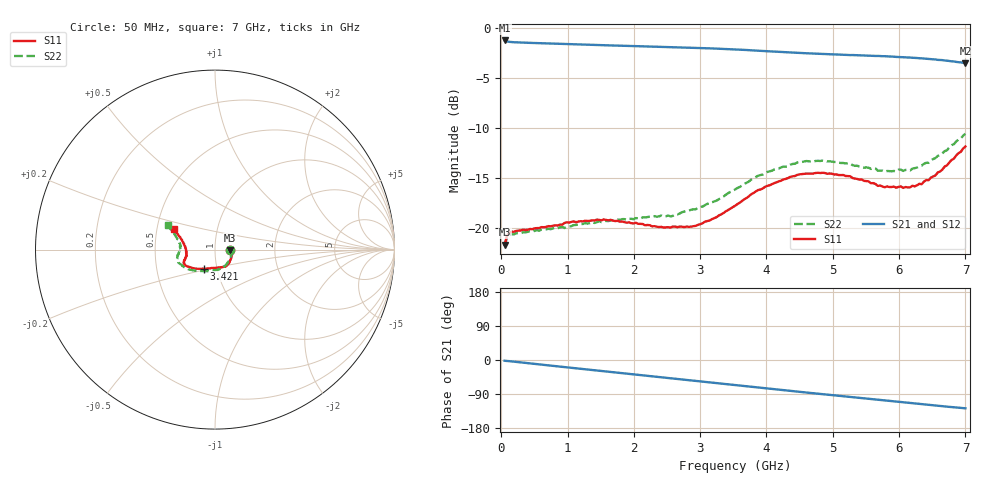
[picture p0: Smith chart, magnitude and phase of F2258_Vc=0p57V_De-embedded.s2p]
! Integrated Device Technology
! Corporate Headquarters
! 6024 Silver Creek Valley Road
! San Jose, CA 95138  USA
! Phone:  1-408-284-8200
! Toll Free:  1-800-223-1366
! Webpage:  http://www.idt.com/
! Timing and RF Division
! 515 Groton Road, Suite 102
! Westford, MA 01886-6024
! Device:  F2258
! Description: Voltage Variable RF Attenuator
! Frequency:  50.0 -  6000.00 MHz
! Package:  3x3 mm Thin QFN Plastic Package: 16 pin
! Ports:  2 RF, 2 DC
!  Pin  1  = NC
!  Pin  2  = NC
!  Pin  3  = RF2  = Port 2
!  Pin  4  = GND
!  Pin  5  = Vdd
!  Pin  6  = NC
!  Pin  7  = VCTRL
!  Pin  8  = NC
!  Pin  9  = GND
!  Pin 10  = RF1  = Port 1
!  Pin 11  = NC
!  Pin 12  = NC
!  Pin 13  = NC
!  Pin 14  = NC
!  Pin 15  = NC
!  Pin 16  = NC
! Vcntrl:  0.570 Volts
! Vdd:  +3.300 Volts
! Current:  1.106 mA
! Data:  The device was measured on a the F2258 evaluation board which has
!  individual transmission lines to the RF pins.  Data was collected
!  using a calibrated network analyzer.  The evaluation board was
!  de-embedded using a TRL calibration technique.
!  The reference plane is the edge of the package pin.
! Misc:  SN 10
!  Action Tracker AT0285
! Date Measured:  2014-12-10
! Date:  2016-01-13  MJV
! Note:
!  Integrated Device Technology supplies this data as a sample of measured
!  data at the package pin for this product.  Your particular data for this
!  product may vary.
!  Data was taken at 25 degrees C.
!  Integrated Device Technology reserves the right to change this data at anytime.
!Freq_(GHz)  S11M_(dB)  S11P_(deg)  S21M_(dB)  S21P_(deg)  S12M_(dB)  S12P_(deg)  S22M_(dB)  S22P_(deg)
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# GHz S dB R 50
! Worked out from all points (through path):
!   201 points, 50 MHz to 7 GHz, reference 50 ohm
!   highest |S21| = -1.21 dB at 50 MHz (marker M1); lowest = -3.5 dB at 7 GHz (marker M2)
!   group delay of S21, straight-line fit = 50.5 ps
!   lowest |S11| = -21.6 dB at 50 MHz (marker M3), VSWR 1.18, Z = 59 - j0.48 ohm
!   |S11| at or under -10 dB: start of sweep to end of sweep
!   |S22| runs from -21.8 to -10.5 dB; largest |S21 - S12| = 0.0006
!   S11 on the Smith chart (normalised r, x): 50 MHz: 1.18, -0.01; 3.421 GHz: 0.86, -0.19; 7 GHz: 0.61, +0.15
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0.05  -21.63 -2.8  -1.21 -2.0  -1.21 -2.0  -21.78 -2.9
0.08475  -20.76 -4.5  -1.30 -2.5  -1.30 -2.5  -20.94 -4.6
0.15425  -20.33 -7.0  -1.37 -3.7  -1.37 -3.7  -20.58 -8.1
0.71025  -19.77 -29.3  -1.51 -14.1  -1.50 -14.1  -20.05 -33.6
1.2315  -19.31 -48.2  -1.61 -23.9  -1.61 -23.9  -19.56 -56.5
1.6485  -19.15 -58.8  -1.70 -31.5  -1.70 -31.5  -19.21 -69.5
2.37825  -19.88 -77.0  -1.83 -44.8  -1.83 -44.8  -18.81 -88.5
2.552  -19.92 -82.4  -1.86 -48.0  -1.87 -48.0  -18.81 -93.7
2.93425  -19.75 -98.4  -1.94 -55.1  -1.94 -55.1  -18.09 -107.5
3.247  -18.88 -112.5  -2.02 -61.0  -2.02 -61.0  -17.23 -119.9
3.42075  -18.17 -120.7  -2.07 -64.3  -2.08 -64.3  -16.48 -127.0
3.525  -17.75 -124.6  -2.11 -66.2  -2.11 -66.2  -16.12 -130.9
4.0115  -15.75 -141.3  -2.28 -75.3  -2.28 -75.3  -14.36 -147.2
4.46325  -14.65 -151.0  -2.44 -83.4  -2.45 -83.4  -13.42 -158.8
4.7065  -14.52 -154.4  -2.52 -87.7  -2.52 -87.7  -13.31 -163.2
5.2625  -14.79 -160.8  -2.67 -97.4  -2.68 -97.4  -13.51 -171.8
5.6795  -15.75 -166.7  -2.75 -104.6  -2.76 -104.6  -14.23 -177.6
5.85325  -15.87 -170.8  -2.81 -107.7  -2.81 -107.7  -14.28 177.7
6.166  -15.90 -179.0  -2.91 -113.3  -2.92 -113.3  -14.21 171.5
6.33975  -15.59 173.9  -2.99 -116.4  -3.00 -116.4  -13.73 167.0
6.6525  -14.13 162.9  -3.17 -121.9  -3.18 -121.9  -12.51 160.0
7  -11.82 153.3  -3.47 -127.4  -3.48 -127.4  -10.54 152.4
